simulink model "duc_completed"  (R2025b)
settings: Solver=VariableStepAuto  StartTime=0.0  StopTime=100  RelTol=1e-3
InitFcn:
  | PreprocIn0data = dataPreProc('data/input_sig_i0.txt');
  | PreprocIn1data = dataPreProc('data/input_sig_i1.txt');
  | PreprocOutdata = dataPreProc('data/output_adder.txt');
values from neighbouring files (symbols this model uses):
  tmp = zeros(1,size(txt{1},1))    [check_sim_output.m]
undefined symbols (not defined in the file or in its folder): adder, aie, code, duc_chain, duc_chain_ipconfig, DUCchain, Evaluation, netlist, Platform, S, Symmetric, VCK190, Versal, vmctmp, vsva2197, xcvc1902
libraries: aieDSP x10, matrix_library x6, aieBasic x4, dspsrcs4 x3, aieUtilities x1, vmcUtilities x1

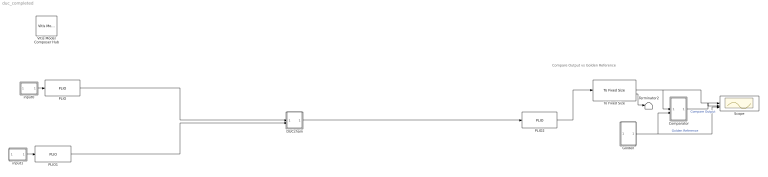
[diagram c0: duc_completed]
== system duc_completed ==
  note: Compare Output vs Golden Reference
  Comparator : Subsystem
  DUCchain : Subsystem
  Golden : Subsystem
  PLIO : aieBasic/PLIO  PlioWidth=64  PlioFreqSpec=off  PlioFreq=250  ColLocation=0  channel=0  blockJsonConstraints=[]  deprecateConstraints=0
  PLIO1 : aieBasic/PLIO  PlioWidth=64  PlioFreqSpec=off  PlioFreq=250  ColLocation=0  channel=0  blockJsonConstraints=[]  deprecateConstraints=0
  PLIO2 : aieBasic/PLIO  PlioWidth=64  PlioFreqSpec=off  PlioFreq=250  ColLocation=0  channel=0  blockJsonConstraints=[]  deprecateConstraints=0
  Scope : Scope  NumInputPorts=3
  Terminator2 : Terminator
  To Fixed Size : aieUtilities/To Fixed Size  Mode=Produce a valid output signal  OutputSize=3072  CopyMethod=Buffer samples to form output  HasStatusOutput=on
  Vitis Model Composer Hub : vmcUtilities/Vitis Model Composer Hub  Tag=genX  CodeGeneration=off  SubsystemName=DUCchain  BlockHierPath=duc_chain/DUCchain  CompilationType=HDLCompilation  SubsystemType=AIENode  ExportTypeV2=IP Catalog  StartColumn=1  NumberOfColumns=1  TargetDirectory=./code  exportDesign=off  analyzeDesign=on  validateDesignOnHw=off  ExportType=AI Engines  IpVendor=xilinx.com  IpLibrary=hls  IpVersion=1.0  IpHWLanguage=Verilog  AieCompilerOptions={}  AieSimulatorOptions={}  CreateTestbench=on  TestbenchStackSize=10  RunRtlSim=off  RunCSim=off  RunAieSim=off  AieSimTimeout=50000  RunAieSimProfiling=off  LaunchVitisAnalyzer=off  PlotOutput=off  RunX86Sim=off  X86SimTimeout=10  GenHwImage=off  GenLibadfXo=off  GenHwValidationCode=off  PlatformType=Specify Platform  Platform=/opt/amd/2025.2/Vitis/base_platforms/xilinx_vck190_base_202520_1/xilinx_vck190_base_202520_1.xpfm  HwSystemType=Baremetal  HwValidationTarget=hw  ProjDevice=Versal VCK190 Evaluation Platform (xcvc1902-vsva2197-2MP-e-S)  ProjDevicePart=xcvc1902-vsva2197-2MP-e-S  AIEType=AIE  SamplePeriod=-1  ClockFrequency=200  DataPathParallelism=1  xilinxfamily=versalaicore  part=xcvc1902  speed=-2MP-e-S  package=vsva2197  directory=./netlist  testbench=off  incr_netlist=off  synthesis_tool=Vivado  clock_wrapper=Clock Enables  dbl_ovrd=According to Block Masks  dcm_input_clock_period=10  sysclk_period=10  simulink_period=1  eval_field=0  IPInfoJsonString="{\"DUTSubsystemName\":\"DUCchain\",\"AIESubsystem\":{\"SubsystemName\":\"DUCchain\",\"TargetDirectory\":\"./code\",\"AIEArrayConfig\":\"Use entire AIE array\",\"StartColumn\":\"0\",\"NumberOfColumns\":\"1\"},\"SubsystemTag\":\"AIENode\"}"  LogFileName=/home/amd/training/vmc_duc/lab/code/model_composer.log  NThreads=4  IPConfigFile=/tmp/vmctmp-14207516001596194974/duc_chain_ipconfig.json
  input0 : Subsystem
  input1 : Subsystem
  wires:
  input0/1(Out1) -> PLIO/1
  input1/1(Out1) -> PLIO1/1
  To Fixed Size/1 -> Scope/1, Comparator/1(In1)
  To Fixed Size/2 -> Terminator2/1
  Golden/1(Out1) -> Comparator/2(In2), Scope/3  "Golden Reference"
  Comparator/1(Out1) -> Scope/2  "Compare Output"
  PLIO2/1 -> To Fixed Size/1
  PLIO/1 -> DUCchain/1(In1)
  PLIO1/1 -> DUCchain/2(In2)
  DUCchain/1(Out1) -> PLIO2/1

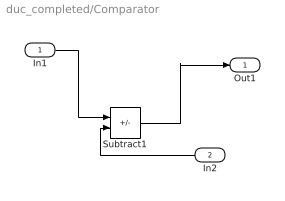
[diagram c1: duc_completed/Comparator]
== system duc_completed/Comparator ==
  In1 : Inport
  In2 : Inport  Port=2
  Subtract1 : Sum  Inputs=+-  OutDataTypeStr=double
  Out1 : Outport
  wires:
  In1/1 -> Subtract1/1
  In2/1 -> Subtract1/2
  Subtract1/1 -> Out1/1

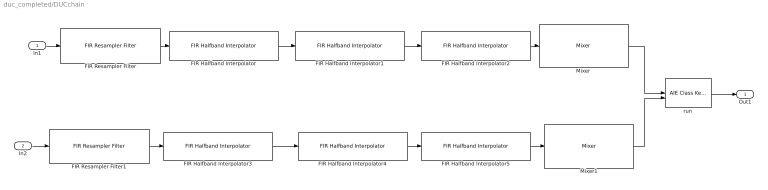
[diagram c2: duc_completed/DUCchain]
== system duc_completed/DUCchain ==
  In1 : Inport
  In2 : Inport  Port=2
  FIR Halfband Interpolator : aieDSP/FIR Halfband Interpolator  data_type=cint16  coef_type=int16  use_coeff_reload=off  dual_ip=off  num_outputs=off  coeff=[90, -522, 1814, -5208, 20212, 32767]  fir_length=31  input_window_size=384  shift_val=15  rnd_mode=Round symmetrical to infinity  sat_mode=3-Symmetric  interp_poly=1  upshift_ct=off  casc_length=1  AIE_VARIANT=1  TP_API=0  ssr=1  blockJsonConstraints=[]  blockJsonConstraintsInternal=[]  spec=vmc_fir_interpolate_hb.json  SerializedMaskParamNames=[]  SerializedMaskParamValues=[]  SerializedMaskParamVisibilities=[]  block_type=FIR Halfband Interpolator  SerializedMaskParamDataypes=typename|typename|uint|uint|uint|coef_type|uint|uint|uint|uint|uint|uint|uint|uint|uint|uint|uint  SerializedMaskParamEnumStrArr=0|0|0|0|0|0|0|0|0|Floor,Ceiling,Round to positive infinity,Round to negative infinity,Round symmetrical to infinity,Round symmetrical to zero,Round convergent to even,Round convergent to odd|0-None,1-Asymmetric,3-Symmetric|0|0|0|0|0|0  SerializedMaskParamEnumValArr=0|0|0|0|0|0|0|0|0|0,1,2,3,4,5,6,7|0,1,3|0|0|0|0|0|0  SerializedMaskParamVectorArr=0|0|0|0|0|1|0|0|0|0|0|0|0|0|0|0|0  SerializedMaskParamKeys=TT_DATA|TT_COEFF|TP_USE_COEFF_RELOAD|TP_DUAL_IP|TP_NUM_OUTPUTS|coeff|TP_FIR_LEN|TP_INPUT_WINDOW_VSIZE|TP_SHIFT|TP_RND|TP_SAT|TP_PARA_INTERP_POLY|TP_UPSHIFT_CT|TP_CASC_LEN|AIE_VARIANT|TP_API|TP_SSR
  FIR Halfband Interpolator1 : aieDSP/FIR Halfband Interpolator  data_type=cint16  coef_type=int16  use_coeff_reload=off  dual_ip=off  num_outputs=off  coeff=[479, -3461, 19366, 32767]  fir_length=31  input_window_size=768  shift_val=15  rnd_mode=Round symmetrical to infinity  sat_mode=3-Symmetric  interp_poly=1  upshift_ct=off  casc_length=1  AIE_VARIANT=1  TP_API=0  ssr=1  blockJsonConstraints=[]  blockJsonConstraintsInternal=[]  spec=vmc_fir_interpolate_hb.json  SerializedMaskParamNames=[]  SerializedMaskParamValues=[]  SerializedMaskParamVisibilities=[]  block_type=FIR Halfband Interpolator  SerializedMaskParamDataypes=typename|typename|uint|uint|uint|coef_type|uint|uint|uint|uint|uint|uint|uint|uint|uint|uint|uint  SerializedMaskParamEnumStrArr=0|0|0|0|0|0|0|0|0|Floor,Ceiling,Round to positive infinity,Round to negative infinity,Round symmetrical to infinity,Round symmetrical to zero,Round convergent to even,Round convergent to odd|0-None,1-Asymmetric,3-Symmetric|0|0|0|0|0|0  SerializedMaskParamEnumValArr=0|0|0|0|0|0|0|0|0|0,1,2,3,4,5,6,7|0,1,3|0|0|0|0|0|0  SerializedMaskParamVectorArr=0|0|0|0|0|1|0|0|0|0|0|0|0|0|0|0|0  SerializedMaskParamKeys=TT_DATA|TT_COEFF|TP_USE_COEFF_RELOAD|TP_DUAL_IP|TP_NUM_OUTPUTS|coeff|TP_FIR_LEN|TP_INPUT_WINDOW_VSIZE|TP_SHIFT|TP_RND|TP_SAT|TP_PARA_INTERP_POLY|TP_UPSHIFT_CT|TP_CASC_LEN|AIE_VARIANT|TP_API|TP_SSR
  FIR Halfband Interpolator2 : aieDSP/FIR Halfband Interpolator  data_type=cint16  coef_type=int16  use_coeff_reload=off  dual_ip=off  num_outputs=off  coeff=[-2117, 18499, 32767]  fir_length=31  input_window_size=1536  shift_val=15  rnd_mode=Round symmetrical to infinity  sat_mode=3-Symmetric  interp_poly=1  upshift_ct=off  casc_length=1  AIE_VARIANT=1  TP_API=0  ssr=1  blockJsonConstraints=[]  blockJsonConstraintsInternal=[]  spec=vmc_fir_interpolate_hb.json  SerializedMaskParamNames=[]  SerializedMaskParamValues=[]  SerializedMaskParamVisibilities=[]  block_type=FIR Halfband Interpolator  SerializedMaskParamDataypes=typename|typename|uint|uint|uint|coef_type|uint|uint|uint|uint|uint|uint|uint|uint|uint|uint|uint  SerializedMaskParamEnumStrArr=0|0|0|0|0|0|0|0|0|Floor,Ceiling,Round to positive infinity,Round to negative infinity,Round symmetrical to infinity,Round symmetrical to zero,Round convergent to even,Round convergent to odd|0-None,1-Asymmetric,3-Symmetric|0|0|0|0|0|0  SerializedMaskParamEnumValArr=0|0|0|0|0|0|0|0|0|0,1,2,3,4,5,6,7|0,1,3|0|0|0|0|0|0  SerializedMaskParamVectorArr=0|0|0|0|0|1|0|0|0|0|0|0|0|0|0|0|0  SerializedMaskParamKeys=TT_DATA|TT_COEFF|TP_USE_COEFF_RELOAD|TP_DUAL_IP|TP_NUM_OUTPUTS|coeff|TP_FIR_LEN|TP_INPUT_WINDOW_VSIZE|TP_SHIFT|TP_RND|TP_SAT|TP_PARA_INTERP_POLY|TP_UPSHIFT_CT|TP_CASC_LEN|AIE_VARIANT|TP_API|TP_SSR
  FIR Halfband Interpolator3 : aieDSP/FIR Halfband Interpolator  data_type=cint16  coef_type=int16  use_coeff_reload=off  dual_ip=off  num_outputs=off  coeff=[90, -522, 1814, -5208, 20212, 32767]  fir_length=31  input_window_size=384  shift_val=15  rnd_mode=Round symmetrical to infinity  sat_mode=3-Symmetric  interp_poly=1  upshift_ct=off  casc_length=1  AIE_VARIANT=1  TP_API=0  ssr=1  blockJsonConstraints=[]  blockJsonConstraintsInternal=[]  spec=vmc_fir_interpolate_hb.json  SerializedMaskParamNames=[]  SerializedMaskParamValues=[]  SerializedMaskParamVisibilities=[]  block_type=FIR Halfband Interpolator  SerializedMaskParamDataypes=typename|typename|uint|uint|uint|coef_type|uint|uint|uint|uint|uint|uint|uint|uint|uint|uint|uint  SerializedMaskParamEnumStrArr=0|0|0|0|0|0|0|0|0|Floor,Ceiling,Round to positive infinity,Round to negative infinity,Round symmetrical to infinity,Round symmetrical to zero,Round convergent to even,Round convergent to odd|0-None,1-Asymmetric,3-Symmetric|0|0|0|0|0|0  SerializedMaskParamEnumValArr=0|0|0|0|0|0|0|0|0|0,1,2,3,4,5,6,7|0,1,3|0|0|0|0|0|0  SerializedMaskParamVectorArr=0|0|0|0|0|1|0|0|0|0|0|0|0|0|0|0|0  SerializedMaskParamKeys=TT_DATA|TT_COEFF|TP_USE_COEFF_RELOAD|TP_DUAL_IP|TP_NUM_OUTPUTS|coeff|TP_FIR_LEN|TP_INPUT_WINDOW_VSIZE|TP_SHIFT|TP_RND|TP_SAT|TP_PARA_INTERP_POLY|TP_UPSHIFT_CT|TP_CASC_LEN|AIE_VARIANT|TP_API|TP_SSR
  FIR Halfband Interpolator4 : aieDSP/FIR Halfband Interpolator  data_type=cint16  coef_type=int16  use_coeff_reload=off  dual_ip=off  num_outputs=off  coeff=[479, -3461, 19366, 32767]  fir_length=31  input_window_size=768  shift_val=15  rnd_mode=Round symmetrical to infinity  sat_mode=3-Symmetric  interp_poly=1  upshift_ct=off  casc_length=1  AIE_VARIANT=1  TP_API=0  ssr=1  blockJsonConstraints=[]  blockJsonConstraintsInternal=[]  spec=vmc_fir_interpolate_hb.json  SerializedMaskParamNames=[]  SerializedMaskParamValues=[]  SerializedMaskParamVisibilities=[]  block_type=FIR Halfband Interpolator  SerializedMaskParamDataypes=typename|typename|uint|uint|uint|coef_type|uint|uint|uint|uint|uint|uint|uint|uint|uint|uint|uint  SerializedMaskParamEnumStrArr=0|0|0|0|0|0|0|0|0|Floor,Ceiling,Round to positive infinity,Round to negative infinity,Round symmetrical to infinity,Round symmetrical to zero,Round convergent to even,Round convergent to odd|0-None,1-Asymmetric,3-Symmetric|0|0|0|0|0|0  SerializedMaskParamEnumValArr=0|0|0|0|0|0|0|0|0|0,1,2,3,4,5,6,7|0,1,3|0|0|0|0|0|0  SerializedMaskParamVectorArr=0|0|0|0|0|1|0|0|0|0|0|0|0|0|0|0|0  SerializedMaskParamKeys=TT_DATA|TT_COEFF|TP_USE_COEFF_RELOAD|TP_DUAL_IP|TP_NUM_OUTPUTS|coeff|TP_FIR_LEN|TP_INPUT_WINDOW_VSIZE|TP_SHIFT|TP_RND|TP_SAT|TP_PARA_INTERP_POLY|TP_UPSHIFT_CT|TP_CASC_LEN|AIE_VARIANT|TP_API|TP_SSR
  FIR Halfband Interpolator5 : aieDSP/FIR Halfband Interpolator  data_type=cint16  coef_type=int16  use_coeff_reload=off  dual_ip=off  num_outputs=off  coeff=[-2117, 18499, 32767]  fir_length=31  input_window_size=1536  shift_val=15  rnd_mode=Round symmetrical to infinity  sat_mode=3-Symmetric  interp_poly=1  upshift_ct=off  casc_length=1  AIE_VARIANT=1  TP_API=0  ssr=1  blockJsonConstraints=[]  blockJsonConstraintsInternal=[]  spec=vmc_fir_interpolate_hb.json  SerializedMaskParamNames=[]  SerializedMaskParamValues=[]  SerializedMaskParamVisibilities=[]  block_type=FIR Halfband Interpolator  SerializedMaskParamDataypes=typename|typename|uint|uint|uint|coef_type|uint|uint|uint|uint|uint|uint|uint|uint|uint|uint|uint  SerializedMaskParamEnumStrArr=0|0|0|0|0|0|0|0|0|Floor,Ceiling,Round to positive infinity,Round to negative infinity,Round symmetrical to infinity,Round symmetrical to zero,Round convergent to even,Round convergent to odd|0-None,1-Asymmetric,3-Symmetric|0|0|0|0|0|0  SerializedMaskParamEnumValArr=0|0|0|0|0|0|0|0|0|0,1,2,3,4,5,6,7|0,1,3|0|0|0|0|0|0  SerializedMaskParamVectorArr=0|0|0|0|0|1|0|0|0|0|0|0|0|0|0|0|0  SerializedMaskParamKeys=TT_DATA|TT_COEFF|TP_USE_COEFF_RELOAD|TP_DUAL_IP|TP_NUM_OUTPUTS|coeff|TP_FIR_LEN|TP_INPUT_WINDOW_VSIZE|TP_SHIFT|TP_RND|TP_SAT|TP_PARA_INTERP_POLY|TP_UPSHIFT_CT|TP_CASC_LEN|AIE_VARIANT|TP_API|TP_SSR
  FIR Resampler Filter : aieDSP/FIR Resampler Filter  data_type=cint16  coef_type=int16  use_coeff_reload=off  num_outputs=off  coeff=[-8,-15,2,27,38,-1,-67,-86,1,139,171,-2,-257,-309,2,443,522,-3,-724,-842,4,1144,1324,-4,-1789,-2078,5,2866,3402,-5,-5080,-6495,6,13412,27026,32762,27026,13412,6,-6495,-5080,-5,3402,2866,5,-2078,-1789,-4,1324,1144,4,-842,-724,-3,522,443,2,-309,-257,-2,171,139,1,-86,-67,-1,38,27,2,-15,-8]  fir_length=30  interpolate_factor=3  decimate_factor=2  input_window_size=256  shift_val=15  rnd_mode=Round symmetrical to infinity  sat_mode=3-Symmetric  interp_poly=1  deci_poly=1  casc_length=1  AIE_VARIANT=1  TP_API=0  dual_ip=0  ssr=1  blockJsonConstraints=[]  blockJsonConstraintsInternal=[]  spec=vmc_fir_resampler.json  SerializedMaskParamNames=[]  SerializedMaskParamValues=[]  SerializedMaskParamVisibilities=[]  block_type=FIR Resampler Filter  SerializedMaskParamDataypes=typename|typename|uint|uint|coef_type|uint|uint|uint|uint|uint|uint|uint|uint|uint|uint|uint|uint|uint|uint  SerializedMaskParamEnumStrArr=0|0|0|0|0|0|0|0|0|0|Floor,Ceiling,Round to positive infinity,Round to negative infinity,Round symmetrical to infinity,Round symmetrical to zero,Round convergent to even,Round convergent to odd|0-None,1-Asymmetric,3-Symmetric|0|0|0|0|0|0|0  SerializedMaskParamEnumValArr=0|0|0|0|0|0|0|0|0|0|0,1,2,3,4,5,6,7|0,1,3|0|0|0|0|0|0|0  SerializedMaskParamVectorArr=0|0|0|0|1|0|0|0|0|0|0|0|0|0|0|0|0|0|0  SerializedMaskParamKeys=TT_DATA|TT_COEFF|TP_USE_COEFF_RELOAD|TP_NUM_OUTPUTS|coeff|TP_FIR_LEN|TP_INTERPOLATE_FACTOR|TP_DECIMATE_FACTOR|TP_INPUT_WINDOW_VSIZE|TP_SHIFT|TP_RND|TP_SAT|TP_PARA_INTERP_POLY|TP_PARA_DECI_POLY|TP_CASC_LEN|AIE_VARIANT|TP_API|TP_DUAL_IP|TP_SSR
  FIR Resampler Filter1 : aieDSP/FIR Resampler Filter  data_type=cint16  coef_type=int16  use_coeff_reload=off  num_outputs=off  coeff=[-8,-15,2,27,38,-1,-67,-86,1,139,171,-2,-257,-309,2,443,522,-3,-724,-842,4,1144,1324,-4,-1789,-2078,5,2866,3402,-5,-5080,-6495,6,13412,27026,32762,27026,13412,6,-6495,-5080,-5,3402,2866,5,-2078,-1789,-4,1324,1144,4,-842,-724,-3,522,443,2,-309,-257,-2,171,139,1,-86,-67,-1,38,27,2,-15,-8]  fir_length=30  interpolate_factor=3  decimate_factor=2  input_window_size=256  shift_val=15  rnd_mode=Round symmetrical to infinity  sat_mode=3-Symmetric  interp_poly=1  deci_poly=1  casc_length=1  AIE_VARIANT=1  TP_API=0  dual_ip=0  ssr=1  blockJsonConstraints=[]  blockJsonConstraintsInternal=[]  spec=vmc_fir_resampler.json  SerializedMaskParamNames=[]  SerializedMaskParamValues=[]  SerializedMaskParamVisibilities=[]  block_type=FIR Resampler Filter  SerializedMaskParamDataypes=typename|typename|uint|uint|coef_type|uint|uint|uint|uint|uint|uint|uint|uint|uint|uint|uint|uint|uint|uint  SerializedMaskParamEnumStrArr=0|0|0|0|0|0|0|0|0|0|Floor,Ceiling,Round to positive infinity,Round to negative infinity,Round symmetrical to infinity,Round symmetrical to zero,Round convergent to even,Round convergent to odd|0-None,1-Asymmetric,3-Symmetric|0|0|0|0|0|0|0  SerializedMaskParamEnumValArr=0|0|0|0|0|0|0|0|0|0|0,1,2,3,4,5,6,7|0,1,3|0|0|0|0|0|0|0  SerializedMaskParamVectorArr=0|0|0|0|1|0|0|0|0|0|0|0|0|0|0|0|0|0|0  SerializedMaskParamKeys=TT_DATA|TT_COEFF|TP_USE_COEFF_RELOAD|TP_NUM_OUTPUTS|coeff|TP_FIR_LEN|TP_INTERPOLATE_FACTOR|TP_DECIMATE_FACTOR|TP_INPUT_WINDOW_VSIZE|TP_SHIFT|TP_RND|TP_SAT|TP_PARA_INTERP_POLY|TP_PARA_DECI_POLY|TP_CASC_LEN|AIE_VARIANT|TP_API|TP_DUAL_IP|TP_SSR
  Mixer : aieDSP/Mixer  data_type=cint16  input_window_size=3072  ssr=1  rnd_mode=Round symmetrical to infinity  sat_mode=3-Symmetric  mixer_mode=Single Input Mode  initialPhaseOffset=0  USE_PHASE_RELOAD=off  PHASE_RELOAD_API=off  phase_increment=715827883  phase_increment_reload=off  AIE_VARIANT=1  TP_API=0  blockJsonConstraints=[]  blockJsonConstraintsInternal=[]  spec=vmc_mixer.json  SerializedMaskParamNames=[]  SerializedMaskParamValues=[]  SerializedMaskParamVisibilities=[]  block_type=Mixer  SerializedMaskParamDataypes=typename|uint|uint|uint|uint|uint|uint|uint|uint|uint|uint|uint|uint  SerializedMaskParamEnumStrArr=0|0|0|Floor,Ceiling,Round to positive infinity,Round to negative infinity,Round symmetrical to infinity,Round symmetrical to zero,Round convergent to even,Round convergent to odd|0-None,1-Asymmetric,3-Symmetric|Single Input Mode,Dual Input Mode|0|0|0|0|0|0|0  SerializedMaskParamEnumValArr=0|0|0|0,1,2,3,4,5,6,7|0,1,3|1,2|0|0|0|0|0|0|0  SerializedMaskParamVectorArr=0|0|0|0|0|0|0|0|0|0|0|0|0  SerializedMaskParamKeys=TT_DATA|TP_INPUT_WINDOW_VSIZE|TP_SSR|TP_RND|TP_SAT|TP_MIXER_MODE|initialPhaseOffset|TP_USE_PHASE_RELOAD|TP_PHASE_RELOAD_API|phaseInc|TP_USE_PHASE_INC_RELOAD|AIE_VARIANT|TP_API
  Mixer1 : aieDSP/Mixer  data_type=cint16  input_window_size=3072  ssr=1  rnd_mode=Round symmetrical to infinity  sat_mode=3-Symmetric  mixer_mode=Single Input Mode  initialPhaseOffset=0  USE_PHASE_RELOAD=off  PHASE_RELOAD_API=off  phase_increment=3042268501  phase_increment_reload=off  AIE_VARIANT=1  TP_API=0  blockJsonConstraints=[]  blockJsonConstraintsInternal=[]  spec=vmc_mixer.json  SerializedMaskParamNames=[]  SerializedMaskParamValues=[]  SerializedMaskParamVisibilities=[]  block_type=Mixer  SerializedMaskParamDataypes=typename|uint|uint|uint|uint|uint|uint|uint|uint|uint|uint|uint|uint  SerializedMaskParamEnumStrArr=0|0|0|Floor,Ceiling,Round to positive infinity,Round to negative infinity,Round symmetrical to infinity,Round symmetrical to zero,Round convergent to even,Round convergent to odd|0-None,1-Asymmetric,3-Symmetric|Single Input Mode,Dual Input Mode|0|0|0|0|0|0|0  SerializedMaskParamEnumValArr=0|0|0|0,1,2,3,4,5,6,7|0,1,3|1,2|0|0|0|0|0|0|0  SerializedMaskParamVectorArr=0|0|0|0|0|0|0|0|0|0|0|0|0  SerializedMaskParamKeys=TT_DATA|TP_INPUT_WINDOW_VSIZE|TP_SSR|TP_RND|TP_SAT|TP_MIXER_MODE|initialPhaseOffset|TP_USE_PHASE_RELOAD|TP_PHASE_RELOAD_API|phaseInc|TP_USE_PHASE_INC_RELOAD|AIE_VARIANT|TP_API
  run : aieBasic/AIE Class Kernel  KernelAllAttrs=s[12;12;9;9;19;14;21;23;21;23;24;21;15;17;12;24;26;26;26;27;28;9;21;23;23;23;24;25;14;19;19;29]@FunctionNameDeclFileNamePortNamesPortTypesPortSerializedTypesPortDirectionsPortWindowSizeEnablesPortWindowMarginEnablesPortBufferSizeEnablesPortBufferMarginEnablesPortSynchronicityEnablesPortSignalSizeEnablesPortBufferSizesPortBufferMarginsFunctionDeclFunctionTemplateSpecKindFunctionTemplateParamNamesFu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  PortNames={'mixer_i0'; 'mixer_i1'; 'y'}  PortSerializedTypes={'{Q2{R{Tadf::input_buffer{2{t{Scint16}}{t{Tadf::extents{1{t{}3072}}}}}}}}'; '{Q2{R{Tadf::input_buffer{2{t{Scint16}}{t{Tadf::extents{1{t{}3072}}}}}}}}'; '{Q2{R{Tadf::output_buffer{2{t{Scint16}}{t{Tadf::extents{1{t{}3072}}}}}}}}'}  PortWindowSizes={3.072000000000000000e+03; 3.072000000000000000e+03; 3.072000000000000000e+03}  PortWindowMargins={0.000000000000000000e+00; 0.000000000000000000e+00; 0.000000000000000000e+00}  PortSynchronicities={'sync', 'sync', 'sync'}  PortSignalSizes={0.000000000000000000e+00; 0.000000000000000000e+00; 0.000000000000000000e+00}  ClassTemplateSpecKind=none  ClassTemplateParamNames={}  ClassTemplateParamKinds={}  ClassTemplateParamTypes={}  ClassTemplateParamValues={}  ClassCtorParamNames={}  ClassCtorParamSerializedTypes={}  ClassCtorParamValues={}  ClassIndex=1  ClassCtorIndex=0  ClassTabVisible=on  ClassTemplateParamsVisible=off  ClassCtorDeclVisible=off  ClassCtorParamsVisible=off  FunctionTabVisible=on  FunctionDecl=|  PortAttrs={ 'input', 'mixer_i0', 'adf::input_buffer< cint16, adf::extents< 3072 > > & restrict', '3072', '0', 'sync', ''; 'input', 'mixer_i1', 'adf::input_buffer< cint16, adf::extents< 3072 > > & restrict', '3072', '0', 'sync', ''; 'output', 'y', 'adf::output_buffer< cint16, adf::extents< 3072 > > & restrict', '3072', '', 'sync', '' }  PortAttrsEnables={'off', 'off', 'off', 'off', 'off', 'off', 'off';'off', 'off', 'off', 'off', 'off', 'off', 'off';'off', 'off', 'off', 'off', 'off', 'off', 'off'}  SampleTime=-1  ClassDeclTypeOptions=C[1 1]@t12@class adder;  ClassDecl=class adder;  ClassTemplateParams={}  ClassTemplateParamsEnables={}  ClassCtorDeclTypeOptions=C[1 1]@t7@<empty>  ClassCtorDecl=<empty>  ClassCtorParams={}  KernelHeaderFile=aie/adder.h  KernelClassName=adder  KernelFunction=run  KernelSourceFile=aie/adder.cpp  KernelSearchPaths={}  PreProcOptions={}  blockJsonConstraints=[]
      | void adder::
      | run(adf::input_buffer< cint16, adf::extents< 3072 > > & restrict mixer_i0, adf::input_buffer< cint16, adf::extents< 3072 > > & restrict mixer_i1, adf::output_buffer< cint16, adf::extents< 3072 > > & restrict y)
  Out1 : Outport
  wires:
  FIR Halfband Interpolator1/1 -> FIR Halfband Interpolator2/1
  FIR Resampler Filter1/1 -> FIR Halfband Interpolator3/1
  FIR Halfband Interpolator/1 -> FIR Halfband Interpolator1/1
  Mixer1/1 -> run/2
  FIR Halfband Interpolator3/1 -> FIR Halfband Interpolator4/1
  Mixer/1 -> run/1
  FIR Halfband Interpolator5/1 -> Mixer1/1
  FIR Halfband Interpolator2/1 -> Mixer/1
  FIR Halfband Interpolator4/1 -> FIR Halfband Interpolator5/1
  FIR Resampler Filter/1 -> FIR Halfband Interpolator/1
  run/1 -> Out1/1
  In1/1 -> FIR Resampler Filter/1
  In2/1 -> FIR Resampler Filter1/1

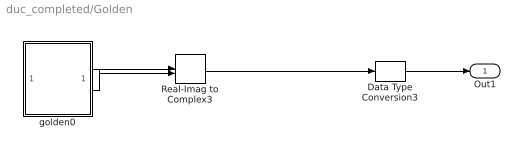
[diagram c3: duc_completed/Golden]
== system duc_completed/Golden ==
  Data Type Conversion3 : DataTypeConversion  OutDataTypeStr=int16
  Real-Imag to Complex3 : RealImagToComplex
  golden0 : Subsystem
  Out1 : Outport
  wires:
  Real-Imag to Complex3/1 -> Data Type Conversion3/1
  golden0/2(Out2) -> Real-Imag to Complex3/2
  golden0/1(Out1) -> Real-Imag to Complex3/1
  Data Type Conversion3/1 -> Out1/1

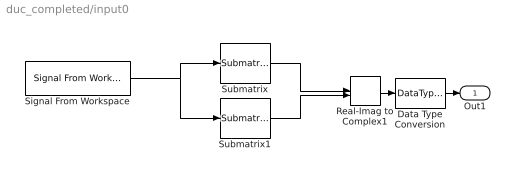
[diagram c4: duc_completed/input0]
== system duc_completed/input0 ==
  Data Type Conversion : DataTypeConversion  OutDataTypeStr=int16
  Real-Imag to Complex1 : RealImagToComplex
  Signal From Workspace : dspsrcs4/Signal From Workspace  X=PreprocIn0data  Ts=1  nsamps=256  OutputAfterFinalValue=Setting to zero  ignoreOrWarnInputAndFrameLengths=off  OutputFrames=off
  Submatrix : matrix_library/Submatrix  RowSpan=All rows  RowStartMode=First  RowStartIndex=1  RowEndMode=Last  RowEndIndex=1  ColSpan=One column  ColStartMode=First  ColStartIndex=1  ColEndMode=Last  ColEndIndex=1
  Submatrix1 : matrix_library/Submatrix  RowSpan=All rows  RowStartMode=First  RowStartIndex=1  RowEndMode=Last  RowEndIndex=1  ColSpan=One column  ColStartMode=Last  ColStartIndex=1  ColEndMode=Last  ColEndIndex=1
  Out1 : Outport
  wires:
  Signal From Workspace/1 -> Submatrix1/1, Submatrix/1
  Submatrix/1 -> Real-Imag to Complex1/1
  Submatrix1/1 -> Real-Imag to Complex1/2
  Real-Imag to Complex1/1 -> Data Type Conversion/1
  Data Type Conversion/1 -> Out1/1

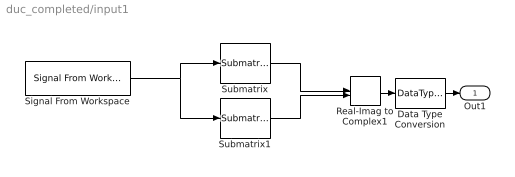
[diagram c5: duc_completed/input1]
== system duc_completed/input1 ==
  Data Type Conversion : DataTypeConversion  OutDataTypeStr=int16
  Real-Imag to Complex1 : RealImagToComplex
  Signal From Workspace : dspsrcs4/Signal From Workspace  X=PreprocIn1data  Ts=1  nsamps=256  OutputAfterFinalValue=Setting to zero  ignoreOrWarnInputAndFrameLengths=off  OutputFrames=off
  Submatrix : matrix_library/Submatrix  RowSpan=All rows  RowStartMode=First  RowStartIndex=1  RowEndMode=Last  RowEndIndex=1  ColSpan=One column  ColStartMode=First  ColStartIndex=1  ColEndMode=Last  ColEndIndex=1
  Submatrix1 : matrix_library/Submatrix  RowSpan=All rows  RowStartMode=First  RowStartIndex=1  RowEndMode=Last  RowEndIndex=1  ColSpan=One column  ColStartMode=Last  ColStartIndex=1  ColEndMode=Last  ColEndIndex=1
  Out1 : Outport
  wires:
  Signal From Workspace/1 -> Submatrix1/1, Submatrix/1
  Submatrix/1 -> Real-Imag to Complex1/1
  Submatrix1/1 -> Real-Imag to Complex1/2
  Real-Imag to Complex1/1 -> Data Type Conversion/1
  Data Type Conversion/1 -> Out1/1

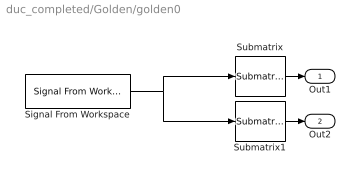
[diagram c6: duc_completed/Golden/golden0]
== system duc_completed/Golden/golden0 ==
  Signal From Workspace : dspsrcs4/Signal From Workspace  X=PreprocOutdata  Ts=1  nsamps=3072  OutputAfterFinalValue=Setting to zero  ignoreOrWarnInputAndFrameLengths=on  OutputFrames=off
  Submatrix : matrix_library/Submatrix  RowSpan=All rows  RowStartMode=First  RowStartIndex=1  RowEndMode=Last  RowEndIndex=1  ColSpan=One column  ColStartMode=First  ColStartIndex=1  ColEndMode=Last  ColEndIndex=1
  Submatrix1 : matrix_library/Submatrix  RowSpan=All rows  RowStartMode=First  RowStartIndex=1  RowEndMode=Last  RowEndIndex=1  ColSpan=One column  ColStartMode=Last  ColStartIndex=1  ColEndMode=Last  ColEndIndex=1
  Out1 : Outport  VectorParamsAs1DForOutWhenUnconnected=off
  Out2 : Outport  Port=2  VectorParamsAs1DForOutWhenUnconnected=off
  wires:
  Submatrix/1 -> Out1/1
  Signal From Workspace/1 -> Submatrix/1, Submatrix1/1
  Submatrix1/1 -> Out2/1
